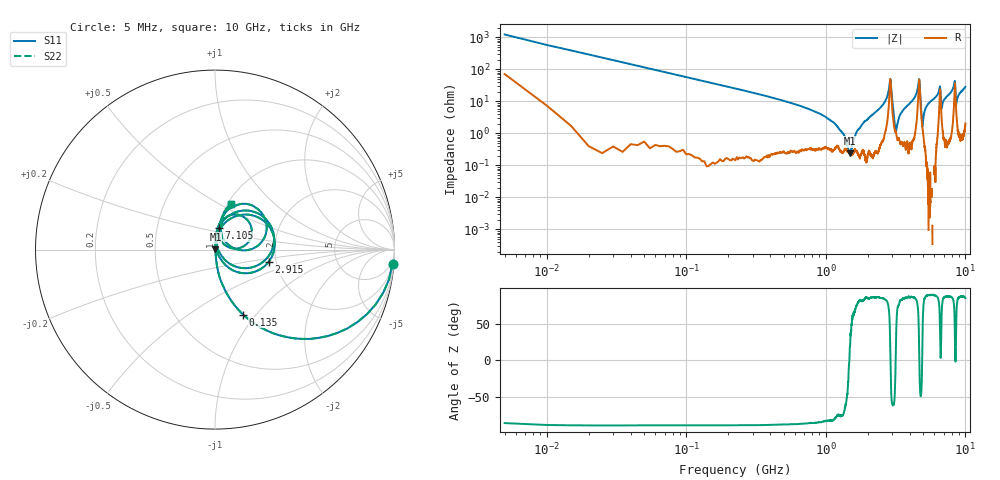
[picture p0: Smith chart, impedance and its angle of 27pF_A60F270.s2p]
! Amotech Co.,Ltd.
! http://www.amotech.co.kr/
! Part Number: A60F270
! These Parameters are Measured in Series Mode Connection
! Operation Temp=25[degC], DC Bias Voltage=0[V]
! Freq. Start=5[MHz] Stop=10[GHz], 2000[Steps]
! Date: Monday, July 20, 2020, 03:38:44
# GHZ S RI R 50.000000
!Freq.(Hz) S11(Real) S11(Imag) S21(Real) S21(Imag) S12(Real) S12(Imag) S22(Real) S22(Imag)
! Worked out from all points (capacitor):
!   2000 points, 5 MHz to 10 GHz, reference 50 ohm
!   read as one part in series: C = 27.2 pF near 55 MHz
!   lowest |Z| = 238 mohm at 1.485 GHz (marker M1)
!   series resonance near 1.476 GHz, so ESL is about 430 pH
!   S11 on the Smith chart (normalised r, x): 5 MHz: 2, -25; 135 MHz: 1.00, -0.86; 2.915 GHz: 1.83, -0.28; 7.105 GHz: 1.01, +0.24; 10 GHz: 1.04, +0.57
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0.005  0.989 -0.0791  0.011 0.0791  0.011 0.0791  0.989 -0.0791
0.065  0.446 -0.4949  0.554 0.4949  0.554 0.4949  0.446 -0.4949
0.135  0.1569 -0.3621  0.8431 0.3621  0.8431 0.3621  0.1569 -0.3621
1.16  0.00365 -0.02  0.9964 0.02  0.9964 0.02  0.00365 -0.02
1.485  0.00227 0.000696  0.9977 -0.000696  0.9977 -0.000696  0.00227 0.000696
1.675  0.00282 0.0115  0.9972 -0.0115  0.9972 -0.0115  0.00282 0.0115
2.83  0.1146 0.1853  0.8854 -0.1853  0.8854 -0.1853  0.1146 0.1853
2.915  0.299 -0.0689  0.701 0.0689  0.701 0.0689  0.299 -0.0689
3.155  0.0117 -0.00276  0.9883 0.00276  0.9883 0.00276  0.0117 -0.00276
3.34  0.00812 0.0294  0.9919 -0.0294  0.9919 -0.0294  0.00812 0.0294
4.41  0.0374 0.1479  0.9626 -0.1479  0.9626 -0.1479  0.0374 0.1479
4.645  0.3076 0.1377  0.6924 -0.1377  0.6924 -0.1377  0.3076 0.1377
4.895  0.0182 -0.00252  0.9818 0.00252  0.9818 0.00252  0.0182 -0.00252
5.005  0.00935 0.0314  0.9906 -0.0314  0.9906 -0.0314  0.00935 0.0314
5.365  0.00684 0.0797  0.9932 -0.0797  0.9932 -0.0797  0.00684 0.0797
6.54  0.1474 0.1882  0.8526 -0.1882  0.8526 -0.1882  0.1474 0.1882
6.67  0.0873 0.00926  0.9127 -0.00926  0.9127 -0.00926  0.0873 0.00926
6.745  0.0336 0.0475  0.9664 -0.0475  0.9664 -0.0475  0.0336 0.0475
7.105  0.0201 0.1182  0.9799 -0.1182  0.9799 -0.1182  0.0201 0.1182
8.335  0.2044 0.247  0.7956 -0.247  0.7956 -0.247  0.2044 0.247
8.59  0.0531 0.0501  0.9469 -0.0501  0.9469 -0.0501  0.0531 0.0501
10  0.0911 0.254  0.9089 -0.254  0.9089 -0.254  0.0911 0.254
